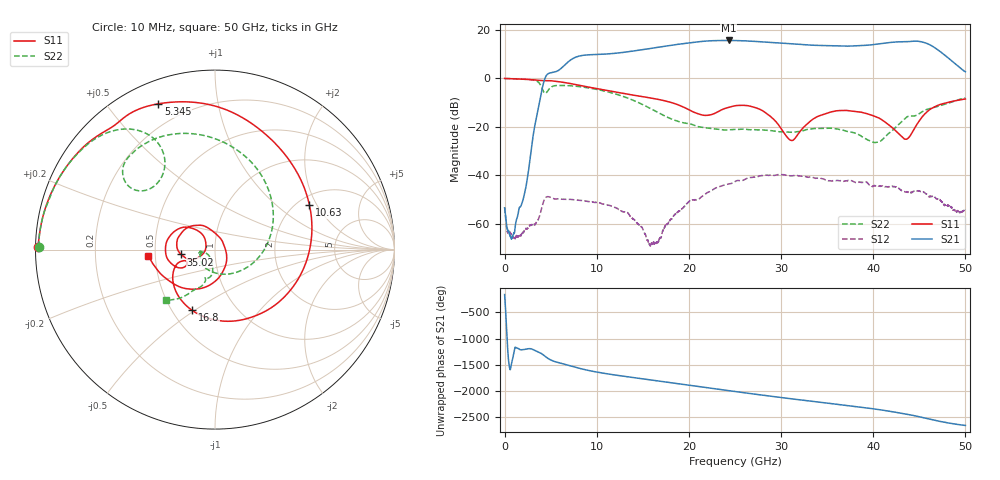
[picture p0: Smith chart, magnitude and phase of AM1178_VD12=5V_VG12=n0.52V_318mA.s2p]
!Keysight Technologies,N5245B,MY58422270,A.16.20.02
!Date: Tuesday, May 26, 2026 20:53:28
!Correction: S11(C  2-Port  )
!S21(C  2-Port  )
!S12(C  2-Port  )
!S22(C  2-Port  )
!S2P File: Measurements: S11, S21, S12, S22:
# Hz S  dB  R 50
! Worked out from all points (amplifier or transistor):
!   6401 points, 10 MHz to 50 GHz, reference 50 ohm
!   highest |S21| = 15.5 dB at 24.3 GHz (marker M1)
!   |S21| within 3 dB of that: 16.35 GHz to 46.68 GHz (30.34 GHz wide, 96.3 % of centre)
!   unconditionally stable (mu >= 1): start of sweep to end of sweep
!   at 8.336 GHz: K = 16.75, MAG = 14.6 dB, |S12| = -50.4 dB
!   at 25 GHz: K = 10.42, MAG = 15.9 dB, |S12| = -42.6 dB
!   at 50 GHz: K = 131.51, MAG = 4.0 dB, |S12| = -53.8 dB
!   S11 on the Smith chart (normalised r, x): 10 MHz: 0.01, +0.01; 5.345 GHz: 0.10, +0.68; 10.63 GHz: 2.31, +1.73; 16.8 GHz: 0.63, -0.49; 35.02 GHz: 0.68, -0.04; 50 GHz: 0.46, -0.04
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1e7  -0.11 179.2  -53.43 -161.5  -53.17 143.7  -0.17 179.1
4.126364e9  -1.01 128.7  -3.62 138.5  -52.14 -99.3  -4.68 118.8
5.34487e9  -1.20 111.2  2.44 7.2  -49.61 -168.9  -3.19 137.4
8.34427e9  -3.13 65.2  9.30 -138.0  -50.38 137.9  -3.58 102.3
1.063288e10  -4.71 25.2  9.87 141.0  -51.83 106.7  -5.12 74.1
1.35776e10  -6.73 -39.0  10.97 65.0  -56.55 72.1  -8.51 30.0
1.667854e10  -8.74 -108.2  12.74 -8.5  -67.49 -63.4  -14.22 -34.0
1.680352e10  -8.83 -110.7  12.81 -11.4  -66.21 122.9  -14.46 -37.1
2.075585e10  -14.34 -160.8  14.86 -105.6  -50.04 155.4  -19.73 -136.6
2.266953e10  -14.72 -151.0  15.45 -153.6  -45.77 143.1  -20.85 -157.0
2.430202e10  -12.02 -160.5  15.54 166.4  -43.62 120.9  -21.29 -163.1
2.5005e10  -11.37 -169.2  15.51 149.4  -42.58 114.3  -21.11 -165.2
2.82153e10  -13.96 141.4  14.91 74.8  -39.93 69.7  -21.39 -173.1
3.076166e10  -24.75 150.3  14.29 18.1  -40.13 33.2  -22.21 -169.5
3.333927e10  -17.21 -155.9  13.59 -36.7  -40.83 5.2  -20.87 -161.7
3.501862e10  -14.36 -171.9  13.37 -72.1  -42.09 -14.4  -20.62 -164.9
3.904125e10  -14.34 138.8  13.49 -158.4  -42.80 -59.7  -24.70 -164.1
4.167354e10  -19.16 100.6  14.65 135.8  -44.66 -92.7  -22.76 -104.7
4.363409e10  -25.10 12.4  15.04 76.4  -46.76 -132.2  -16.03 -101.2
4.533687e10  -15.83 -83.8  14.88 13.9  -46.96 -170.7  -13.77 -108.6
4.703184e10  -11.14 -129.4  11.62 -53.0  -49.84 142.4  -11.58 -118.7
5e10  -8.58 -174.4  2.67 -137.9  -53.82 101.0  -8.12 -134.4
